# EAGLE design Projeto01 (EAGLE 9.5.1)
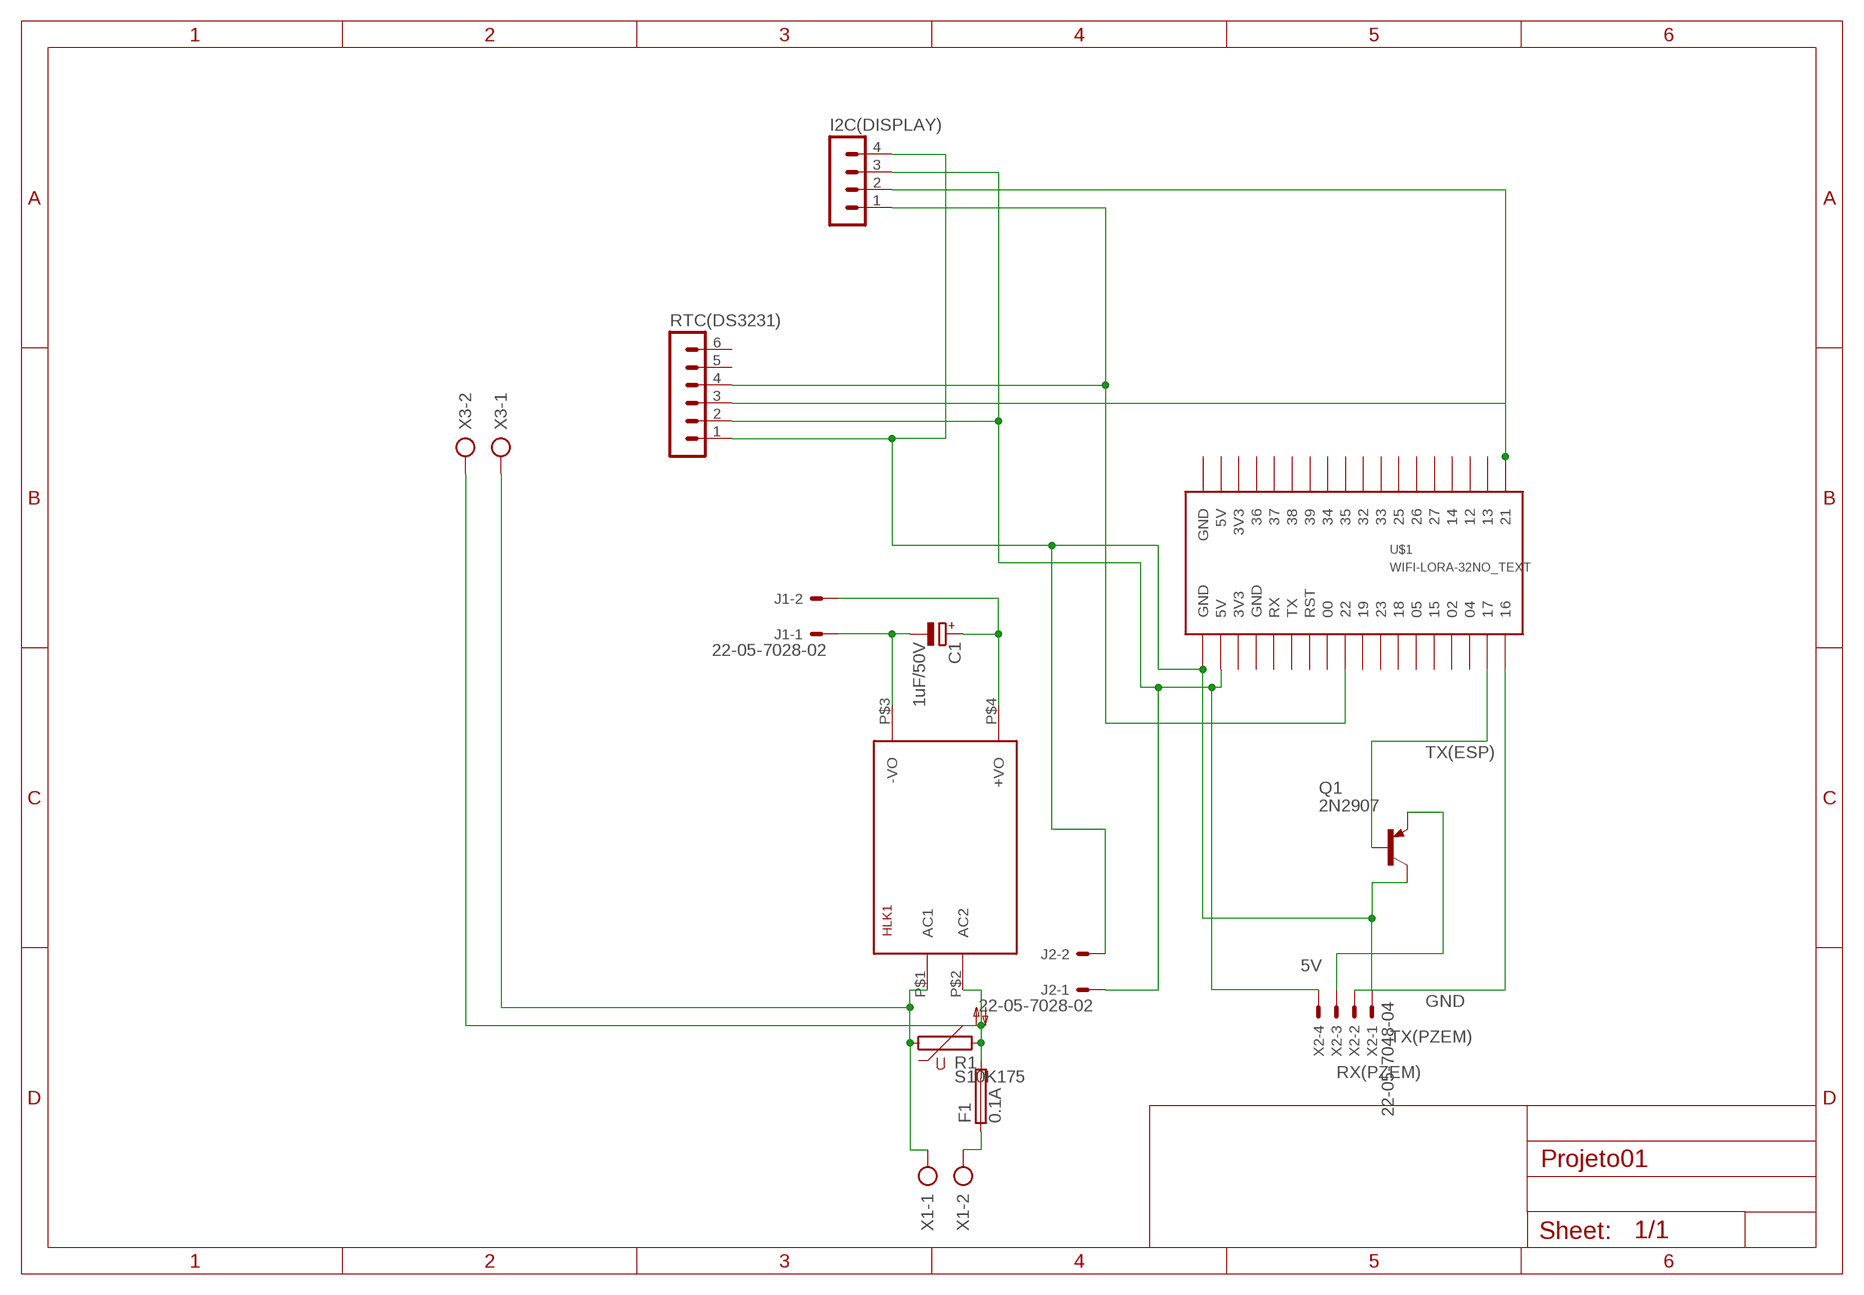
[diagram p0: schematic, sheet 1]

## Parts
C1  1uF/50V  CPOL-EUE2.5-5  [E2,5-5]
F1  0.1A  SH22,5  [SH22,5]
HLK1  HLK-PM013W  [HLK-PM01]
I2C(DISPLAY)  MA04-1  [MA04-1]
J1  22-05-7028-02  [7395-02]
J2  22-05-7028-02  [7395-02]
Q1  2N2907  [TO18]
R1  S10K175  [S10K175]
RTC(DS3231)  MA06-1  [MA06-1]
U$1  WIFI-LORA-32NO_TEXT  [ESP32LORA]
X1  AK500/2-H  [AK500/2-H]
X2  22-05-7048-04  [7395-04]
X3  AK500/2-H  [AK500/2-H]

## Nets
5V: I2C(DISPLAY).3 J2.1 RTC(DS3231).2 U$1.P$2(5V) X2.4
GND: I2C(DISPLAY).4 J2.2 Q1.3(C) RTC(DS3231).1 U$1.P$1(GND) X2.1
N$1: HLK1.P$1(AC1) R1.1 X1.1 X3.1
N$3: F1.1 X1.2
N$4: C1.+ HLK1.P$4(+VO) J1.2
N$5: F1.2 HLK1.P$2(AC2) R1.2 X3.2
N$6: C1.- HLK1.P$3(-VO) J1.1
RX(PZEM): Q1.1(E) X2.3
SCL: I2C(DISPLAY).1 RTC(DS3231).4 U$1.P$9
SDA: I2C(DISPLAY).2 RTC(DS3231).3 U$1.P$19
TX(ESP): Q1.2(B) U$1.P$17
TX(PZEM): U$1.P$18 X2.2
Unconnected: RTC(DS3231).5 RTC(DS3231).6 U$1.P$3(3V3) U$1.P$4(GND) U$1.P$5(RX) U$1.P$6(TX) U$1.P$7(RST) U$1.P$8 U$1.P$10 U$1.P$11 U$1.P$12 U$1.P$13 U$1.P$14 U$1.P$15 U$1.P$16 U$1.P$20 U$1.P$21 U$1.P$22 U$1.P$23 U$1.P$24 U$1.P$25 U$1.P$26 U$1.P$27 U$1.P$28 U$1.P$29 U$1.P$30 U$1.P$31 U$1.P$32 U$1.P$33 U$1.P$34(3V3) U$1.P$35(5V) U$1.P$36(GND)

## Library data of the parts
C1 = rcl:CPOL-EU: POLARIZED CAPACITOR, European symbol; SPICEPREFIX: C
F1 = fuse:SH22,5: FUSE HOLDER; MF: SCHURTER; MPN: 0031.8201; OC_FARNELL: 1162740; OC_NEWARK: 96F8317
HLK1 = HLK-PM01:HLK-PM01: Hi-Link Power Supply HLK-PM01 3W Author: Ahmed Said
I2C(DISPLAY) = con-lstb:MA04-1: PIN HEADER; OC_FARNELL: unknown; OC_NEWARK: unknown
J1 J2 = con-molex:22-?-02: CONNECTOR; MF: MOLEX; OC_FARNELL: 9731601; OC_NEWARK: unknown
Q1 = transistor gabriel:2N2907*: PNP Transistor
R1 = varistor:S10K175: VARISTOR
RTC(DS3231) = con-lstb:MA06-1: PIN HEADER; OC_FARNELL: unknown; OC_NEWARK: unknown
U$1 = ESP32_modules:WIFI-LORA-32
X1 X3 = con-ptr500:AK500/2-H: CONNECTOR; OC_FARNELL: unknown; OC_NEWARK: unknown
X2 = con-molex:22-?-04: CONNECTOR wire to board 2.54 mm (.1 inch) pitch header; MF: MOLEX; OC_FARNELL: unknown; OC_NEWARK: unknown

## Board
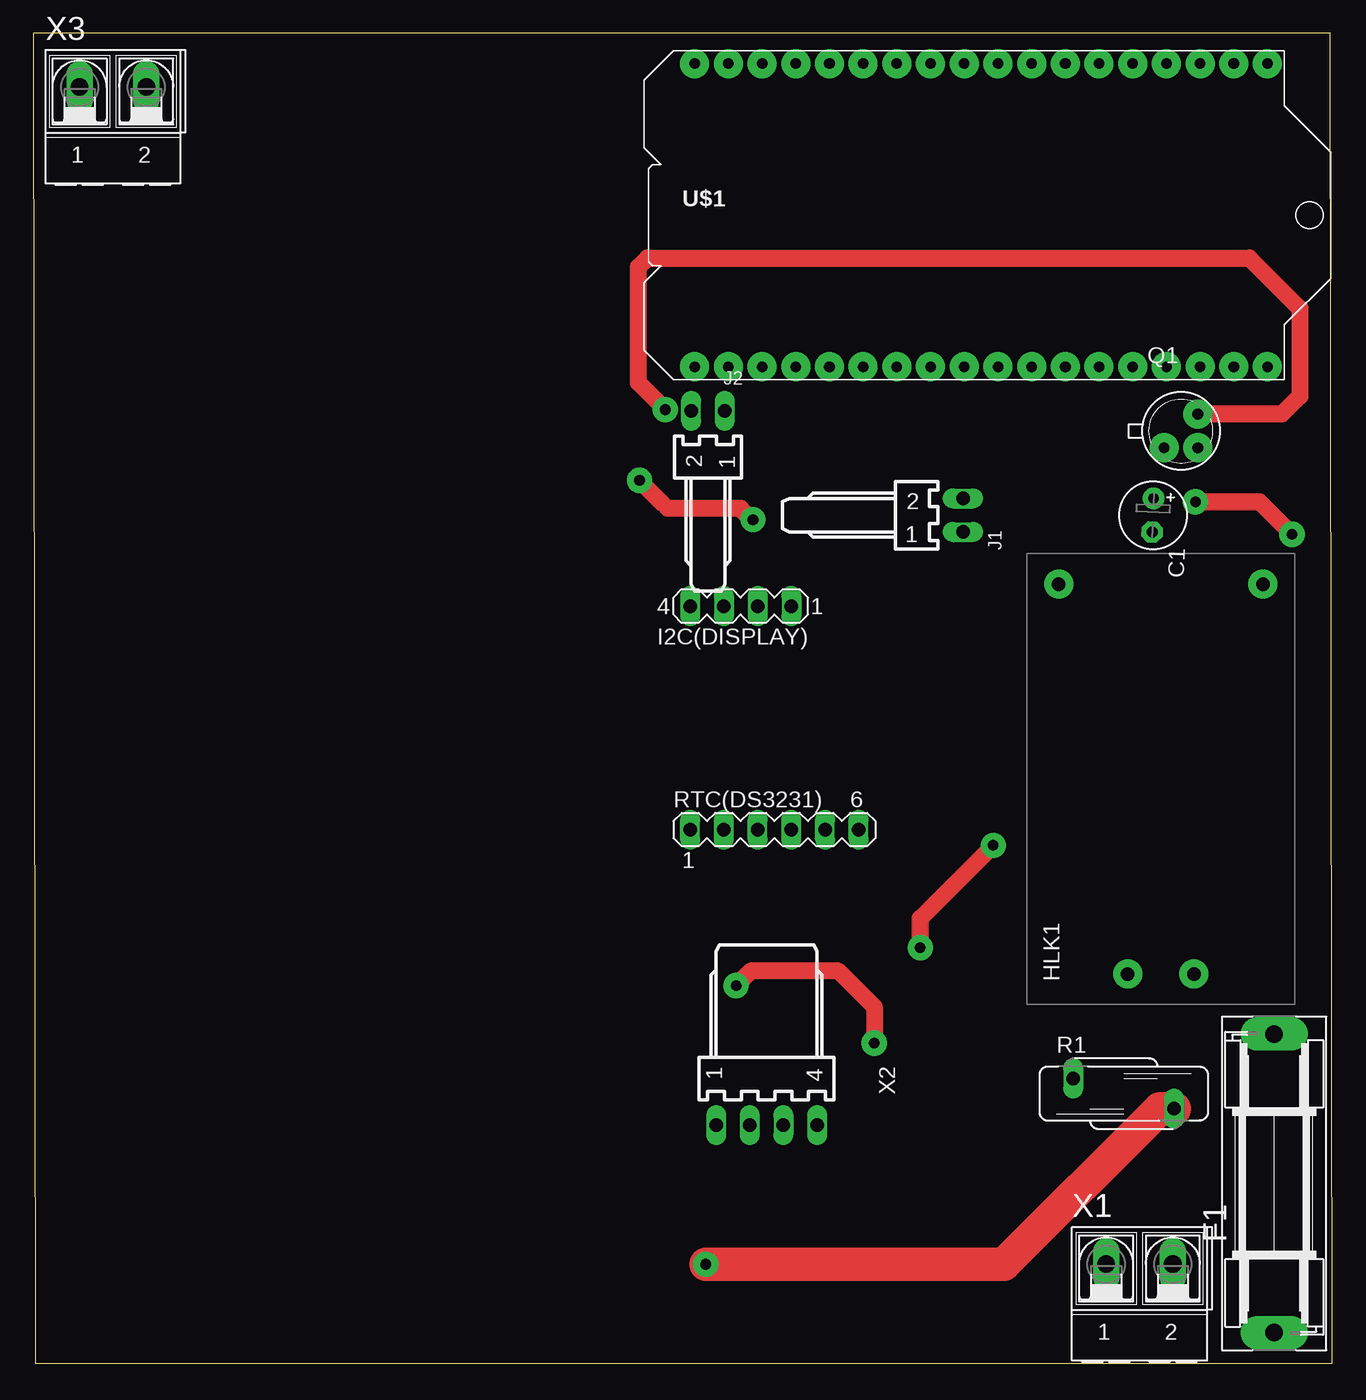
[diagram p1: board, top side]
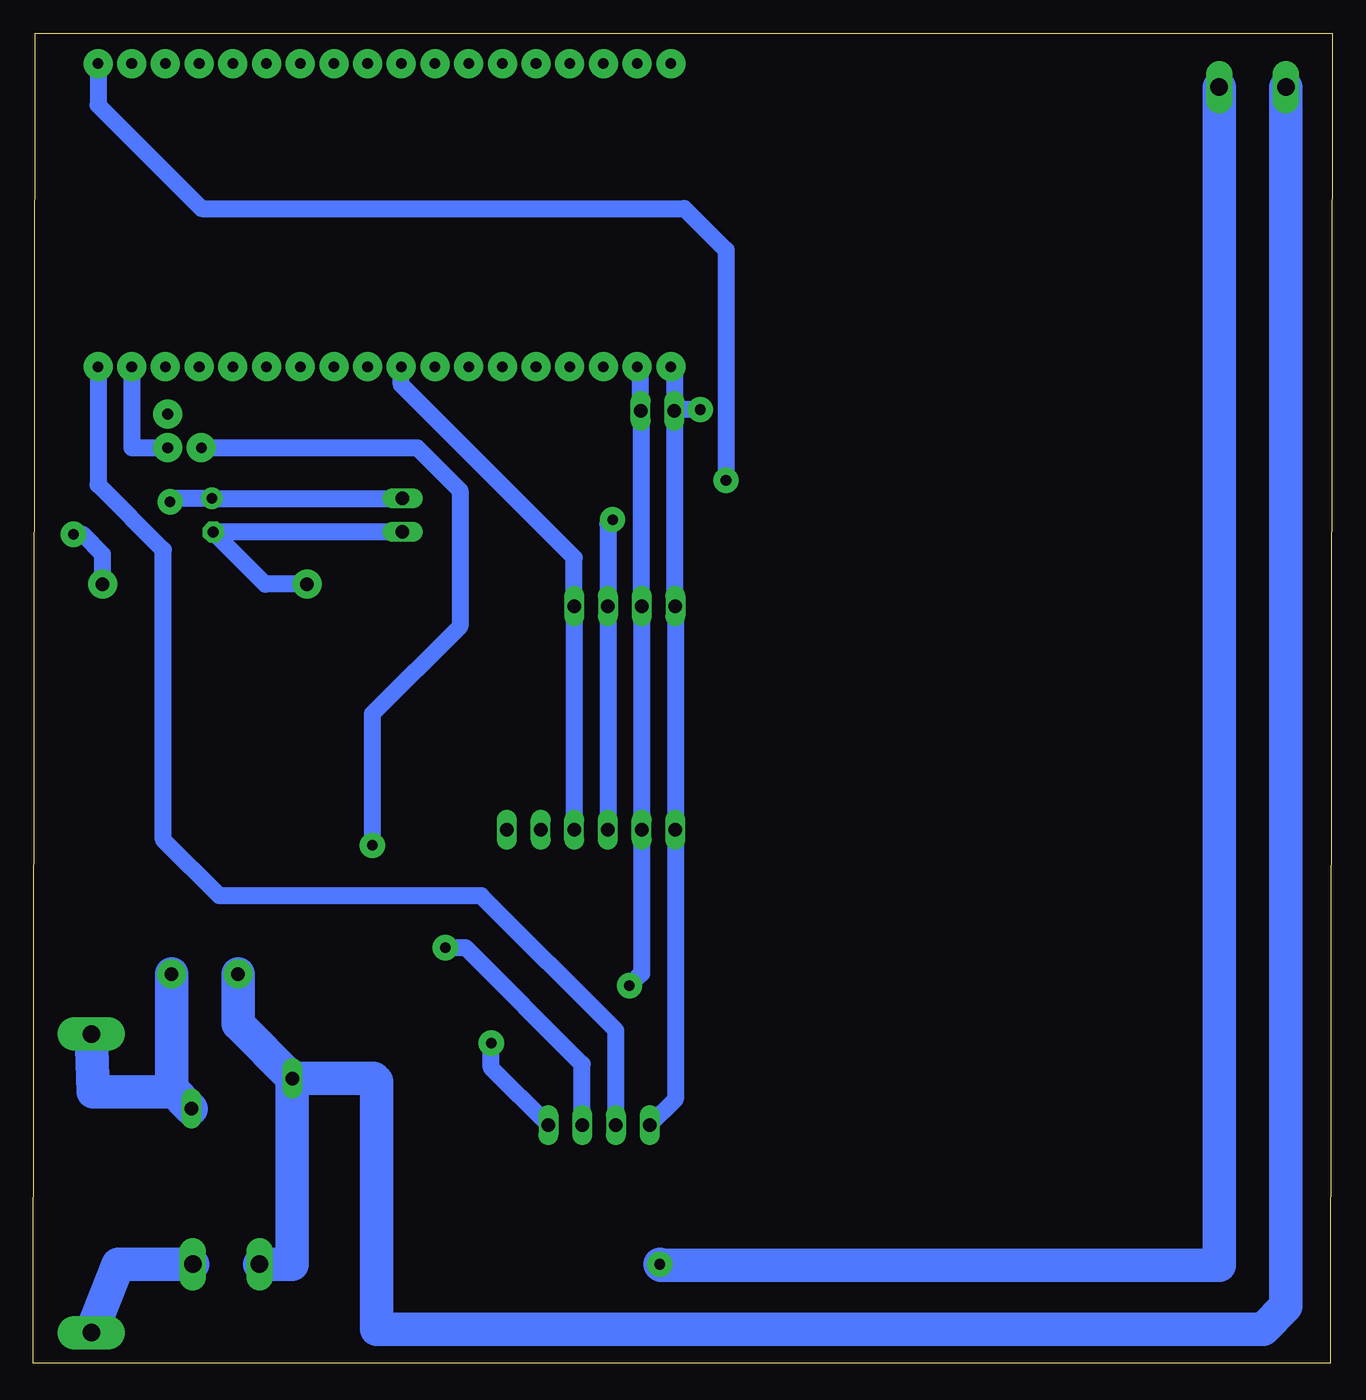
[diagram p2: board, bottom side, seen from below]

Size 97.94 x 100.25 mm. Coordinates in mm from the lower left corner, seen from the top.
Outline: 0.17,0 97.94,0 97.77,100.25 0,100.25 0.17,0
Copper layers (1*16): Top 0.035mm / dielectric 1.5mm / Bottom 0.035mm
Design rules "default": minimum track width 6mil, minimum drill 0.35mm, track to track 6mil, track to pad 6mil, pad to pad 6mil, via to via 6mil, smd to smd 6mil, copper to edge 40mil, drill to drill 6mil, minimum pad ring 10mil, minimum via ring 8mil, stop-mask expansion 4mil, vias tented up to drill 0mil, thermal gap 10mil

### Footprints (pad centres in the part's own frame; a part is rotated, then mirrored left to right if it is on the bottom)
E2,5-5 = drill 0.813 pad 1.6: + -1.27,0 | drill 0.813 pad 1.6 octagon: - 1.27,0
SH22,5 = drill 1.321 pad 2.54 long: 1 -11.252,0; 2 11.252,0
HLK-PM01 = drill 1.016 pad 2.184: P$1 -14.7,2.5; P$2 -14.7,-2.5; P$3 14.7,7.7; P$4 14.7,-7.7
MA04-1 = drill 1.016 long: 1 -3.81,0; 2 -1.27,0; 3 1.27,0; 4 3.81,0
7395-02 = drill 1.016 long: 1 1.27,0; 2 -1.27,0
TO18 = drill 0.813 pad 2.184: 1 -1.27,-1.27; 2 1.27,-1.27; 3 1.27,1.27
S10K175 = drill 1.016 long: 1 -1.143,-3.81; 2 1.143,3.81
MA06-1 = drill 1.016 long: 1 -6.35,0; 2 -3.81,0; 3 -1.27,0; 4 1.27,0; 5 3.81,0; 6 6.35,0
ESP32LORA = drill 0.8 pad 2.184: P$1 -20.32,-11.43; P$2 -17.78,-11.43; P$3 -15.24,-11.43; P$4 -12.7,-11.43; P$5 -10.16,-11.43; P$6 -7.62,-11.43; P$7 -5.08,-11.43; P$8 -2.54,-11.43; P$9 0,-11.43; P$10 2.54,-11.43; P$11 5.08,-11.43; P$12 7.62,-11.43; P$13 10.16,-11.43; P$14 12.7,-11.43; P$15 15.24,-11.43; P$16 17.78,-11.43; P$17 20.32,-11.43; P$18 22.86,-11.43; P$19 22.86,11.43; P$20 20.32,11.43; P$21 17.78,11.43; P$22 15.24,11.43; P$23 12.7,11.43; P$24 10.16,11.43; P$25 7.62,11.43; P$26 5.08,11.43; P$27 2.54,11.43; P$28 0,11.43; P$29 -2.54,11.43; P$30 -5.08,11.43; P$31 -7.62,11.43; P$32 -10.16,11.43; P$33 -12.7,11.43; P$34 -15.24,11.43; P$35 -17.78,11.43; P$36 -20.32,11.43
AK500/2-H = drill 1.321 long: 1 -2.515,0; 2 2.515,0
7395-04 = drill 1.016 long: 1 3.81,0; 2 1.27,0; 3 -1.27,0; 4 -3.81,0

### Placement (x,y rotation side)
C1  84.41,63.92 267.8 top
F1  93.56,13.55 90 top
HLK1  85,44.03 90 top
I2C(DISPLAY)  53.34,57.07 180 top
J1  70.09,63.92 270 top
J2  50.87,71.79 0 top
Q1  86.53,70.27 0 top
R1  82.21,20.32 270 top
RTC(DS3231)  55.88,40.22 0 top
U$1  70.19,86.53 0 top
X1  83.4,7.45 0 top
X2  55.28,17.95 180 top
X3  6.01,96.18 0 top

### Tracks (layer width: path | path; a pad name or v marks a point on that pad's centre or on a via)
5V  (via drill 0.8 pad 1.9)
  Top 1.27: v52.99,28.45 54.09,29.55 60.69,29.55 63.4,26.84 v63.4,24.13
  Bottom 0.152: 52.14,74.83 U$1.P$2 | 52.07,71.72 J2.1 | RTC(DS3231).2
  Bottom 1.27: v63.4,24.13 63.4,22.26 X2.4 | J2.1 | J2.1 52.14,74.83 | 52.07,71.72 I2C(DISPLAY).3 RTC(DS3231).2 | RTC(DS3231).2 52.07,29.37 v52.99,28.45
GND  (via drill 0.8 pad 1.9)
  Top 1.27: v47.66,71.88 45.62,73.91 45.62,82.63 46.3,83.3 91.68,83.3 95.49,79.49 95.49,72.89 94.14,71.54 Q1.3
  Bottom 0.152: RTC(DS3231).1 | 49.52,71.88 J2.2 | 49.6,57.14 I2C(DISPLAY).4
  Bottom 1.27: I2C(DISPLAY).4 RTC(DS3231).1 | RTC(DS3231).1 49.53,19.9 X2.1 | v47.66,71.88 49.52,71.88 | U$1.P$1 49.6,74.83 J2.2 49.6,57.14
N$1
  Bottom 0.152: 72.26,21.46 72.05,21.25
  Bottom 2.54: HLK1.P$1 82.5,25.57 R1.1 | R1.1 78.4,7.45 X1.1 | 72.05,21.25 72.05,2.54 5.22,2.54 3.5,4.27 X3.1 | R1.1 72.26,21.46
N$3
  Bottom 2.54: X1.2 91.52,7.45 F1.1
N$4  (via drill 0.8 pad 1.9)
  Top 1.27: v87.62,64.93 92.44,64.93 v94.9,62.48
  Bottom 0.152: C1.+
  Bottom 1.27: v87.62,64.93 87.36,65.19 C1.+ | v94.9,62.48 94.22,62.48 92.7,60.96 HLK1.P$4 | C1.+ J1.2
N$5  (via drill 0.8 pad 1.9)
  Top 2.54: v50.7,7.45 73.19,7.45 84.92,19.18 R1.2
  Bottom 2.54: HLK1.P$2 87.5,20.66 R1.2 87.29,20.45 93.4,20.45 F1.2 | X3.2 8.53,7.37 50.62,7.37 v50.7,7.45
N$6
  Bottom 0.152: C1.-
  Bottom 1.27: J1.1 C1.- 80.43,58.73 HLK1.P$3
RX(PZEM)  (via drill 0.8 pad 1.9)
  Top 1.27: v66.87,31.32 66.87,33.52 v72.38,39.03
  Bottom 1.27: X2.3 56.55,22.53 65.35,31.32 v66.87,31.32 | Q1.1 69,69 65.77,65.78 65.77,55.54 72.38,48.93 v72.38,39.03
SCL
  Bottom 0.152: RTC(DS3231).4
  Bottom 1.27: U$1.P$9 70.19,73.75 57.15,60.71 I2C(DISPLAY).1 RTC(DS3231).4
SDA  (via drill 0.8 pad 1.9)
  Top 0.152: 47.4,64.85 47.83,64.42 | 54.18,63.58 v54.26,63.58
  Top 1.27: v45.71,66.54 47.4,64.85 | 54.18,63.58 53.33,64.42 47.83,64.42
  Bottom 0.152: RTC(DS3231).3
  Bottom 1.27: U$1.P$19 93.05,94.83 85.24,87.03 48.84,87.03 45.71,83.9 v45.71,66.54 | v54.26,63.58 54.61,63.23 I2C(DISPLAY).2 RTC(DS3231).3
TX(ESP)
  Bottom 1.27: U$1.P$17 90.51,69 Q1.2
TX(PZEM)
  Bottom 1.27: X2.2 54.01,25.07 64.17,35.22 83.89,35.22 88.12,39.45 88.12,61.29 93.05,66.22 U$1.P$18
